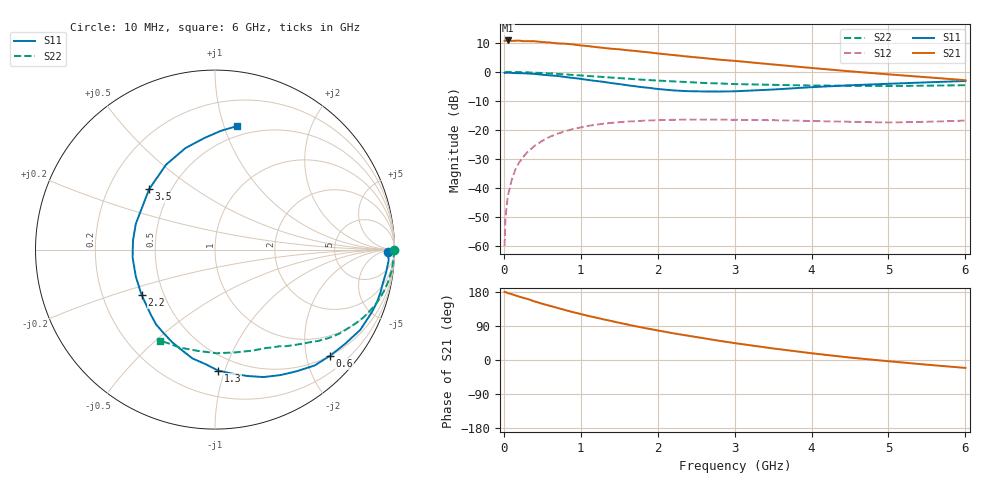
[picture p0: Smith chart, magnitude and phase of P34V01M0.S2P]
! SIEMENS Small Signal Semiconductors
! BFP181
! Si NPN RF Bipolar Junction Transistor in SOT143
! VCE = 4 V  IC = 1 mA
! Common Emitter S-Parameters:  March  1996
# GHz  S  MA  R  50
!  f  S11  S21  S12  S22
! GHz  MAG  ANG  MAG  ANG  MAG  ANG  MAG  ANG
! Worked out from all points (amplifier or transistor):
!   36 points, 10 MHz to 6 GHz, reference 50 ohm
!   highest |S21| = 10.8 dB at 50 MHz (marker M1)
!   |S21| within 3 dB of that: start of sweep to 1.477 GHz
!   unconditionally stable (mu >= 1): 3.163 GHz to end of sweep
!   at 250 MHz: K = 0.10, MSG = 20.0 dB, |S12| = -29.3 dB
!   at 1.4 GHz: K = 0.49, MSG = 12.8 dB, |S12| = -17.5 dB
!   at 6 GHz: K = 1.26, MAG = 3.9 dB, |S12| = -16.8 dB
!   lowest NFmin = 1.30 dB at 450 MHz
!   S11 on the Smith chart (normalised r, x): 10 MHz: 45, -18; 600 MHz: 0.50, -2.47; 1.3 GHz: 0.38, -0.95; 2.2 GHz: 0.38, -0.25; 3.5 GHz: 0.38, +0.34; 6 GHz: 0.41, +1.10
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0.01  0.9625 -0.9  3.438 179.6  0.001 90.9  0.9979 -0.2
0.02  0.9651 -1.4  3.444 179.4  0.003 86.9  0.9946 -0.7
0.05  0.9694 -3.5  3.484 176.9  0.0071 91.4  0.9973 -1.7
0.1  0.9622 -7.3  3.419 173.8  0.0135 84.0  0.9948 -3.4
0.2  0.9522 -14.6  3.462 167.2  0.0278 80.8  0.9917 -6.7
0.25  0.9488 -18.0  3.386 164.1  0.0341 77.6  0.9867 -8.4
0.4  0.9248 -28.9  3.375 154.6  0.0534 71.0  0.9714 -13.3
0.6  0.8721 -42.7  3.205 142.9  0.0767 61.8  0.9425 -19.3
0.8  0.8172 -56.0  3.06 131.6  0.0956 54.0  0.9081 -24.7
0.9  0.7879 -62.6  2.977 126.2  0.1041 50.0  0.8875 -27.4
1.1  0.727 -75.6  2.782 116.2  0.118 43.0  0.8503 -32.0
1.3  0.6744 -88.5  2.59 107.1  0.1286 36.8  0.817 -36.2
1.5  0.619 -101.8  2.454 98.1  0.1364 31.6  0.7817 -39.8
1.8  0.5459 -121.8  2.229 85.6  0.1442 24.8  0.7353 -44.7
2.2  0.481 -148.2  1.955 70.6  0.1498 17.0  0.6875 -50.8
2.8  0.4597 173.6  1.627 50.7  0.1509 8.5  0.6338 -59.3
3  0.464 161.9  1.551 44.6  0.1497 6.1  0.6185 -62.3
3.5  0.498 137.5  1.344 30.5  0.1478 2.1  0.5998 -69.9
4  0.5464 119.9  1.171 17.8  0.1429 -0.7  0.5837 -78.9
4.5  0.5892 106.2  1.024 6.4  0.1385 -2.1  0.5776 -89.0
5.5  0.6619 87.3  0.81 -12.4  0.1385 0.9  0.5801 -110.0
6  0.6983 80.0  0.721 -20.9  0.1452 1.6  0.5909 -121.0
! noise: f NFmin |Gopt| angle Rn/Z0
0.45  1.3  0.7  18  0.5
0.9  1.4  0.6  39  0.52
1.8  1.85  0.4  81  0.47
